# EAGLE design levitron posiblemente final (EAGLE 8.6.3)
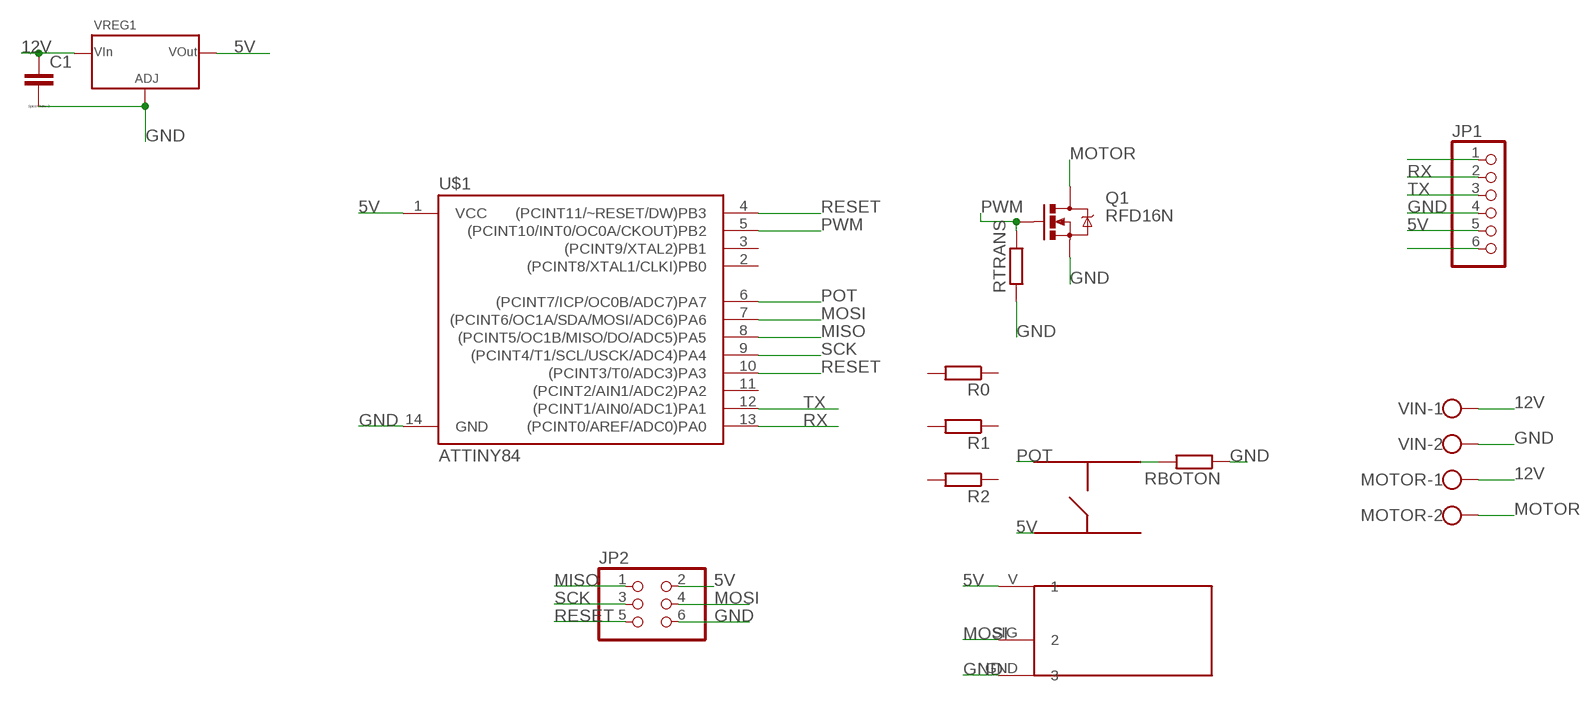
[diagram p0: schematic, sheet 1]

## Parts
C1  CC1206  [C1206]
FC1  POTF  [PAQUETOTE]
JP1  PINHD-1X6  [1X06]
JP2  PINHD-2X3  [2X03]
MOTOR  W237-102  [W237-102]
Q1  RFD16N  [DPACK]
R0  R-EU_R1206  [R1206]
R1  R-EU_R1206  [R1206]
R2  R-EU_R1206  [R1206]
RBOTON  R-EU_R1206  [R1206]
RTRANS  R-EU_R1206  [R1206]
S1  TACTSWITCH  [TACT]
U$1  ATTINY84  [SO14]
VIN  W237-102  [W237-102]
VREG1  ZLDO711  [SOT223]

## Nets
5V: FC1.V JP1.5 JP2.2 S1.3 U$1.1(VCC) VREG1.P$2(VOUT) VREG1.TAB(VOUT)
12V: C1.1 MOTOR.1 VIN.1 VREG1.P$3(VIN)
GND: C1.2 FC1.GND JP1.4 JP2.6 Q1.3(S) RBOTON.1 RTRANS.1 U$1.14(GND) VIN.2 VREG1.P$1(ADJ)
MISO: JP2.1 U$1.8((PCINT5/OC1B/MISO/DO/ADC5)PA5)
MOSI: FC1.SIG JP2.4 U$1.7((PCINT6/OC1A/SDA/MOSI/ADC6)PA6)
MOTOR: MOTOR.2 Q1.2(D)
N$23: RBOTON.2 S1.2
N$24: JP1.1
N$29: JP1.6
POT: S1.1 U$1.6((PCINT7/ICP/OC0B/ADC7)PA7)
PWM: Q1.1(G) RTRANS.2 U$1.5((PCINT10/INT0/OC0A/CKOUT)PB2)
RESET: JP2.5 U$1.4((PCINT11/~RESET/DW)PB3) U$1.10((PCINT3/T0/ADC3)PA3)
RX: JP1.2 U$1.13((PCINT0/AREF/ADC0)PA0)
SCK: JP2.3 U$1.9((PCINT4/T1/SCL/USCK/ADC4)PA4)
TX: JP1.3 U$1.12((PCINT1/AIN0/ADC1)PA1)
Unconnected: R0.1 R0.2 R1.1 R1.2 R2.1 R2.2 S1.4 U$1.2((PCINT8/XTAL1/CLKI)PB0) U$1.3((PCINT9/XTAL2)PB1) U$1.11((PCINT2/AIN1/ADC2)PA2)

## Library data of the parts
C1 = eagle-ltspice:C: CAPACITOR, European symbol; SPICEMODEL: NONE; SPICEPREFIX: C
FC1 = Franco:POTF
JP1 = pinhead:PINHD-1X6: PIN HEADER
JP2 = pinhead:PINHD-2X3: PIN HEADER
MOTOR VIN = con-wago-500:W237-102: WAGO SCREW CLAMP; MPN: 237-102; OC_FARNELL: unknown; OC_NEWARK: 70K9898
Q1 = oliver:RFD16N
R0 R1 R2 RBOTON RTRANS = resistor:R-EU_: RESISTOR, European symbol
S1 = oliver:TACTSWITCH
U$1 = SparkFun-DigitalIC:ATTINY84: Atmel 14-pin 2/4/8kB flash uC; PROD_ID: IC-11285
VREG1 = oliver:ZLDO711: Voltage Regulator for 3.3v or 5v @ 1A depdngin on device, with input supplies up to 18v

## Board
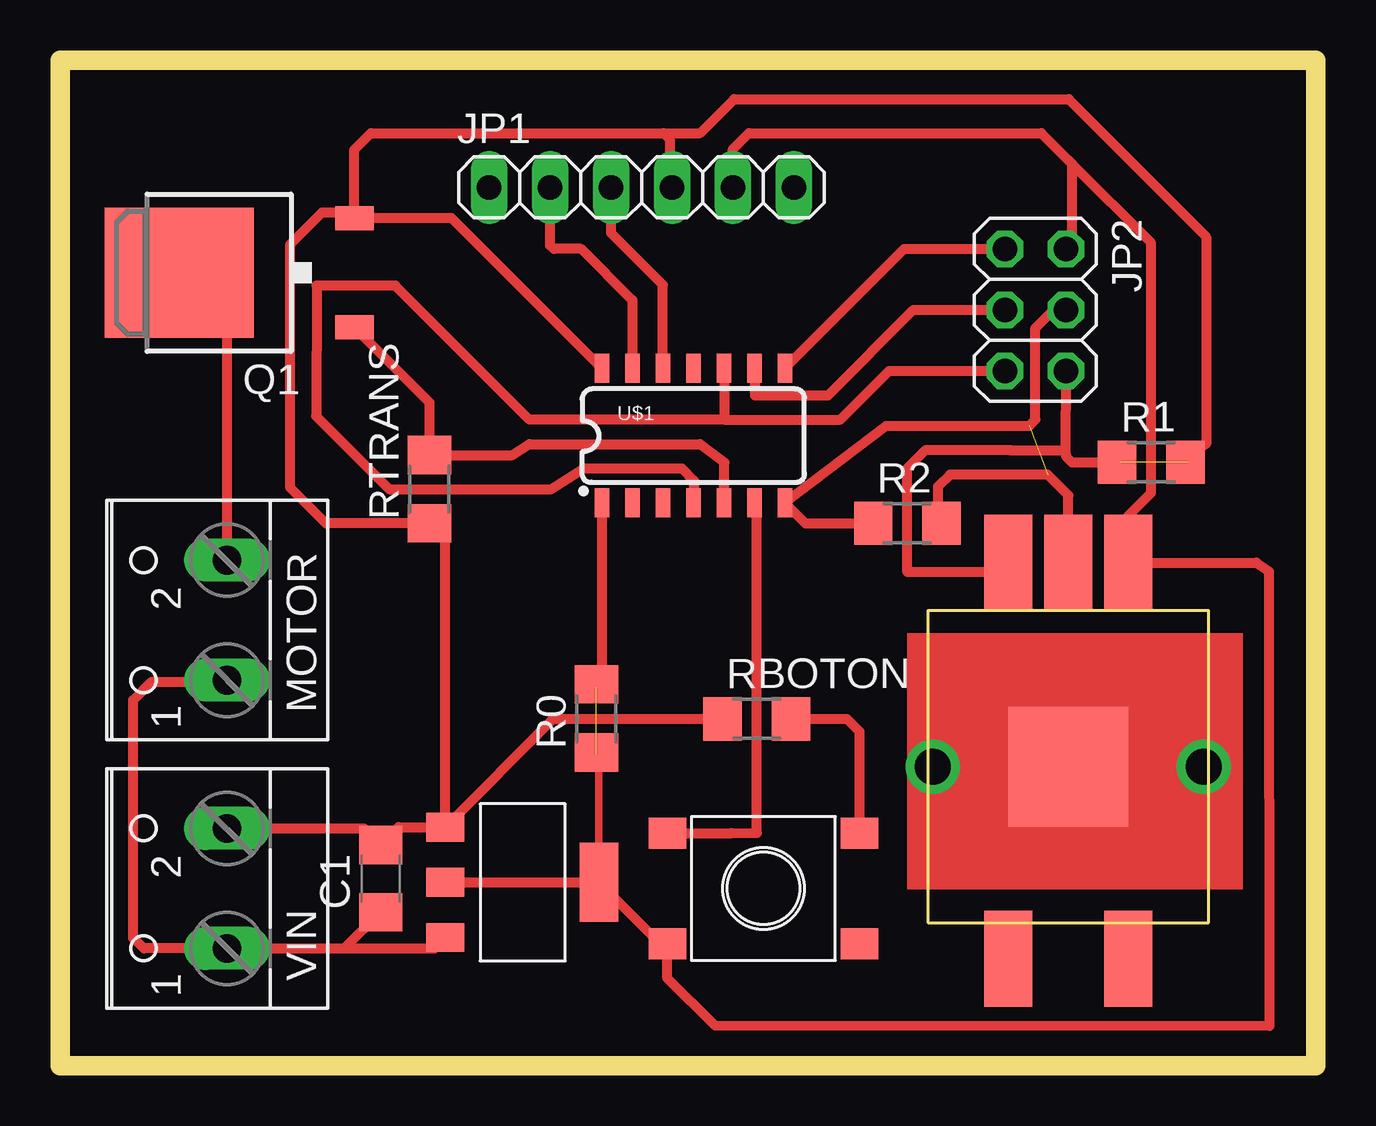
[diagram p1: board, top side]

Size 52.32 x 41.91 mm. Coordinates in mm from the lower left corner, seen from the top.
Outline: 0,0 52.32,0 52.32,41.91 0,41.91 0,0
Copper layers (1*16): Top 0.035mm / dielectric 1.5mm / Bottom 0.035mm
Design rules "default *": minimum track width 10mil, minimum drill 0.35mm, track to track 10mil, track to pad 10mil, pad to pad 10mil, via to via 10mil, smd to smd 6mil, copper to edge 40mil, drill to drill 6mil, minimum pad ring 10mil, minimum via ring 8mil, stop-mask expansion 4mil, vias tented up to drill 0mil, thermal gap 10mil

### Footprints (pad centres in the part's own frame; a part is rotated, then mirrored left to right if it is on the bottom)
C1206 = smd 1.6 x 1.8: 1 -1.4,0; 2 1.4,0
PAQUETOTE = smd 2 x 4: GND 2.5,-8.5; N/A -2.5,8; NO 2.5,8; SIG 0,-8.5; V -2.5,-8.5 | drill 1.5: P$7 -5.65,0; P$8 5.65,0 | smd 5 x 5: PEGA 0,0
1X06 = drill 1.016 long: 1 -6.35,0; 2 -3.81,0; 3 -1.27,0; 4 1.27,0; 5 3.81,0; 6 6.35,0
2X03 = drill 1.016 octagon: 1 -2.54,-1.27; 2 -2.54,1.27; 3 0,-1.27; 4 0,1.27; 5 2.54,-1.27; 6 2.54,1.27
W237-102 = drill 1.194 long: 1 -2.5,-1.27; 2 2.5,-1.27
DPACK = smd 1 x 1.6: 1 -2.28,-4.8; 3 2.28,-4.8 | smd 5.4 x 6.2: 2 0,2.5
R1206 = smd 1.6 x 1.803: 1 -1.422,0; 2 1.422,0
TACT = smd 1.55 x 1.3: 1 -4,2.3; 2 4,2.3; 3 -4,-2.3; 4 4,-2.3
SO14 = smd 0.6 x 1.2: 1 -3.81,-2.8; 2 -2.54,-2.8; 3 -1.27,-2.8; 4 0,-2.8; 5 1.27,-2.8; 6 2.54,-2.8; 7 3.81,-2.8; 8 3.81,2.8; 9 2.54,2.8; 10 1.27,2.8; 11 0,2.8; 12 -1.27,2.8; 13 -2.54,2.8; 14 -3.81,2.8
SOT223 = smd 1.2 x 1.6: P$1 -2.3,-6.4; P$2 0,-6.4; P$3 2.3,-6.4 | smd 3.3 x 1.6: TAB 0,0

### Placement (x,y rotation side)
C1  13.36,7.8 90 top
FC1  42.01,12.47 180 top
JP1  24.23,36.6 0 top
JP2  40.64,31.5 270 top
MOTOR  5.69,18.57 90 top
Q1  7.47,33.05 90 top
R0  22.35,14.48 90 top
R1  45.47,25.15 0 top
R2  35.31,22.61 0 top
RBOTON  29.03,14.45 0 top
RTRANS  15.39,24.03 90 top
S1  29.31,7.39 0 top
U$1  26.39,26.26 0 top
VIN  5.69,7.39 90 top
VREG1  22.45,7.65 270 top

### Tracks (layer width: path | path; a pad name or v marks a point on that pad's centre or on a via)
5V  (1 unrouted)
  Top 0.305: 25.01,5.09 S1.3 | 44.45,20.32 44.45,20.91 FC1.V 44.51,22.92 | 42.16,34.29 JP2.2 | VREG1.TAB 22.45,12.85 22.35,12.95 | 22.58,15.98 22.35,15.75
  Top 0.406: VREG1.P$2 VREG1.TAB 25.01,5.09 | JP1.5 28.04,38.2 28.7,38.86 40.89,38.86 42.04,37.72 42.16,37.59 | 42.16,37.59 42.16,34.29 | U$1.1 22.58,15.98 | S1.3 25.31,3.64 27.31,1.68 50.39,1.65 50.37,20.6 49.84,20.97 FC1.V | 44.51,22.92 45.47,23.88 45.47,34.29 42.16,37.59
12V
  Top 0.305: 15.6,4.89 VREG1.P$3 | 7.62,16 7.02,16 MOTOR.1
  Top 0.406: 11.85,4.89 VIN.1 3.49,4.89 3.05,5.33 3.05,15.24 3.81,16 7.02,16 | 11.85,4.89 C1.1 | 11.85,4.89 15.6,4.89
GND  (1 unrouted)
  Top 0.305: 12.67,9.89 C1.2 14.11,9.95 | Q1.3 12.27,35.56 | 25.4,36.7 JP1.4 | 16.05,21.95 RTRANS.1 | 47.75,25.91 46.99,25.15 | FC1.GND 39.11,20.57
  Top 0.406: VIN.2 12.67,9.89 | 14.11,9.95 VREG1.P$1 | VREG1.P$1 20.56,14.45 RBOTON.1 | 25.15,38.86 12.95,38.86 12.27,38.18 12.27,35.56 10.92,35.56 9.6,34.24 9.6,24.08 11.07,22.61 RTRANS.1 | 25.15,38.86 25.4,38.61 25.4,36.7 | U$1.14 16.32,35.32 Q1.3 | VREG1.P$1 16.05,21.95 | 25.15,38.86 26.67,38.86 28.09,40.28 42.04,40.28 47.75,34.54 47.75,25.91 | JP2.6 41.89,25.65 | 41.89,25.65 41.91,25.4 42.16,25.15 44.2,25.15 | 41.89,25.65 39.6,25.65 39.51,25.67 36.08,25.67 35.31,24.89 35.31,20.57 39.11,20.57
MISO
  Top 0.406: U$1.8 35.17,34.04 JP2.1
MOSI  (1 unrouted)
  Top 0.406: JP2.4 41.4,31.5 40.64,30.73 40.64,26.92 40.39,26.67 34.42,26.67 U$1.7 31.06,22.61 33.78,22.61 | FC1.SIG 42.01,23.77 41.15,24.64 37.08,24.64 36.58,24.13 36.58,22.61
MOTOR
  Top 0.305: 6.96,31.05 Q1.2
  Top 0.406: MOTOR.2 6.96,31.05
N$23
  Top 0.406: RBOTON.2 32.79,14.45 33.31,13.93 S1.2
POT
  Top 0.305: 29.03,23.03 U$1.6
  Top 0.406: S1.1 27.98,9.69 29.03,9.7 29.03,23.03
PWM
  Top 0.305: 27.69,25.15 27.66,25.12
  Top 0.406: Q1.1 15.39,27.64 RTRANS.2 18.85,25.45 19.56,25.91 26.67,25.91 27.69,25.15 | 27.66,25.12 U$1.5
RESET
  Top 0.305: U$1.10 27.69,29.04 | 26.42,23.49 U$1.4
  Top 0.406: 27.69,29.04 27.69,26.92 | 27.69,26.92 32.51,26.92 34.54,28.96 JP2.5 | 27.69,26.92 19.56,26.92 13.97,32.51 10.69,32.51 10.67,27.08 13.72,24.03 20.47,24.03 21.84,24.89 25.91,24.89 26.42,24.38 26.42,23.49
RX
  Top 0.406: U$1.13 23.85,31.9 21.72,34.04 20.57,34.04 20.42,34.19 JP1.2
SCK
  Top 0.305: U$1.9 28.96,29.04
  Top 0.406: 28.96,29.04 28.96,27.94 32,27.94 35.56,31.5 JP2.3
TX
  Top 0.406: U$1.12 25.12,32.54 22.96,34.7 JP1.3
(copper drawn outside any net)
  shapes: Top area x1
